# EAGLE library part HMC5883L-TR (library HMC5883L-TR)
HONEYWELL - HMC5883L-TR - IC, DIGITAL COMPASS, 3 AXIS, 16 PIN Source: Datasheet
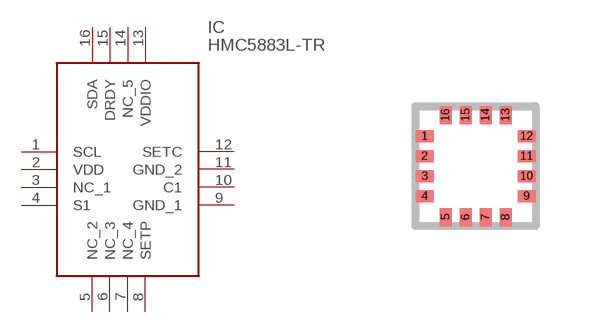
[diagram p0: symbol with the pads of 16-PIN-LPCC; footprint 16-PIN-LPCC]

Designator prefix IC

## HMC5883L-TR (Description: HONEYWELL - HMC5883L-TR - IC, DIGITAL COMPASS, 3 AXIS, 16 PIN; Height: mm; Manufacturer_Name: Honeywell; Manufacturer_Part_Number: HMC5883L-TR; Mouser_Part_Number: N/A; Mouser_Price-Stock: https://www.mouser.co.uk/ProductDetail/Honeywell/HMC5883L-TR?qs=hKcDQsDv3HZv3lHHlqlacQ%3D%3D)  [16-PIN-LPCC]
1  SCL
2  VDD
3  NC_1
4  S1
5  NC_2
6  NC_3
7  NC_4
8  SETP
9  GND_1
10  C1
11  GND_2
12  SETC
13  VDDIO
14  NC_5
15  DRDY
16  SDA

## Footprint 16-PIN-LPCC (pad centres in mm)
16-PIN-LPCC
smd 0.45 x 0.3: 1 -1.275,0.75; 2 -1.275,0.25; 3 -1.275,-0.25; 4 -1.275,-0.75; 9 1.275,-0.75; 10 1.275,-0.25; 11 1.275,0.25; 12 1.275,0.75
smd 0.3 x 0.45: 5 -0.75,-1.275; 6 -0.25,-1.275; 7 0.25,-1.275; 8 0.75,-1.275; 13 0.75,1.275; 14 0.25,1.275; 15 -0.25,1.275; 16 -0.75,1.275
